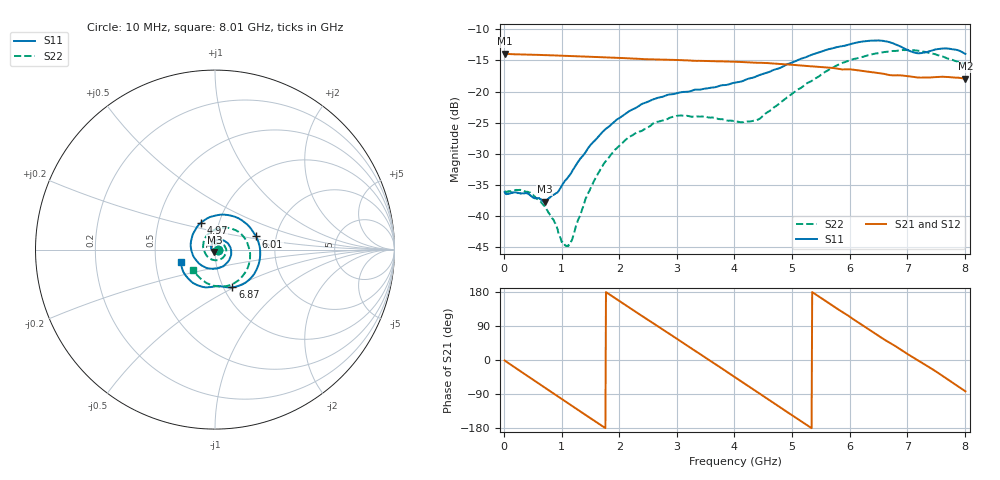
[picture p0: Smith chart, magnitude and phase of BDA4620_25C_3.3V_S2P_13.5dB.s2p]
!Agilent Technologies,E5071B,MY42404982,A.09.10
!Date: Wed May 06 08:51:24 2026
!Data & Calibration Information:
!Freq	S11:SOLT2(ON)	S21:SOLT2(ON)	S12:SOLT2(ON)	S22:SOLT2(ON)
# Hz S RI R 50
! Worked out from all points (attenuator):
!   801 points, 10 MHz to 8.01 GHz, reference 50 ohm
!   highest |S21| = -13.93 dB at 10 MHz (marker M1); lowest = -17.9 dB at 8.01 GHz (marker M2)
!   lowest |S11| = -37.7 dB at 710 MHz (marker M3), VSWR 1.03, Z = 49.7 - j1.26 ohm
!   |S11| at or under -10 dB: start of sweep to end of sweep
!   |S22| runs from -44.8 to -13.3 dB; largest |S21 - S12| = 0.00085
!   S11 on the Smith chart (normalised r, x): 10 MHz: 1.03, -0.00; 4.97 GHz: 0.82, +0.25; 6.01 GHz: 1.57, +0.24; 6.87 GHz: 1.10, -0.49; 8.01 GHz: 0.68, -0.10
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1e7  0.0155 -0.00109  0.2011 -0.00428  0.2014 -0.00435  0.0158 -0.000695
4.4e8  0.00888 -0.0119  0.1385 -0.1414  0.1387 -0.1416  0.0136 -0.00721
7.1e8  -0.00314 -0.0126  0.0565 -0.1879  0.0565 -0.1883  0.00696 -0.00954
1.09e9  -0.0199 0.00143  -0.0726 -0.1795  -0.0728 -0.1797  -0.00471 -0.0033
1.17e9  -0.0212 0.00718  -0.0968 -0.1668  -0.0971 -0.167  -0.00629 -0.000533
1.35e9  -0.0213 0.0209  -0.1432 -0.1271  -0.1434 -0.1272  -0.00834 0.0072
1.59e9  -0.0115 0.0393  -0.181 -0.0565  -0.1812 -0.0565  -0.0063 0.0193
1.9e9  0.0161 0.0543  -0.1816 0.0452  -0.1819 0.0452  0.00617 0.0322
2.31e9  0.0616 0.0424  -0.1045 0.1509  -0.1047 0.151  0.0329 0.0335
2.68e9  0.0894 -0.000193  0.00628 0.1806  0.00657 0.1809  0.0543 0.018
3.39e9  0.0338 -0.0981  0.1688 0.0518  0.1692 0.0515  0.0462 -0.0428
4.01e9  -0.0877 -0.0787  0.1216 -0.1238  0.1217 -0.124  -0.0228 -0.0533
4.41e9  -0.1339 0.00767  0.0122 -0.1696  0.012 -0.17  -0.0585 -0.0106
4.97e9  -0.0787 0.1498  -0.1308 -0.0996  -0.131 -0.0997  -0.0396 0.085
5.35e9  0.0361 0.1949  -0.1593 0.0026  -0.1594 0.0026  0.0299 0.1186
6.01e9  0.2291 0.073  -0.0596 0.1385  -0.0598 0.1388  0.1691 0.0587
6.35e9  0.2473 -0.0659  0.0276 0.1413  0.0277 0.1415  0.1953 -0.0245
6.68e9  0.168 -0.1856  0.0932 0.099  0.0935 0.0992  0.1769 -0.1134
6.87e9  0.0971 -0.21  0.118 0.066  0.1182 0.066  0.1465 -0.1565
7.19e9  0.0156 -0.2023  0.1296 -0.00319  0.13 -0.00312  0.0634 -0.2035
7.56e9  -0.0851 -0.2029  0.1058 -0.0781  0.106 -0.0782  -0.0377 -0.1901
8.01e9  -0.1882 -0.0697  0.0162 -0.1259  0.0164 -0.1262  -0.1212 -0.1125
